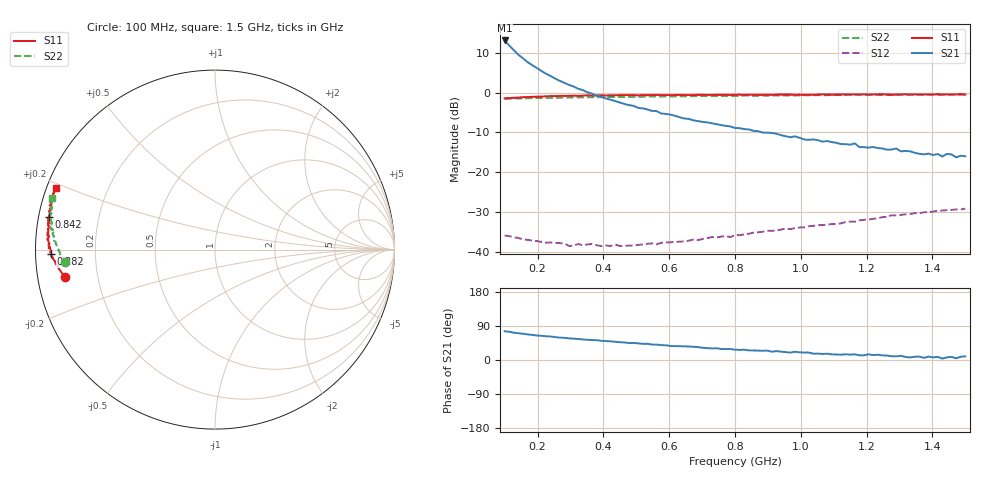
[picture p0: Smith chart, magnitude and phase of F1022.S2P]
!  POLYFET RF DEVICES
!  F1022
!  S PARAMETERS
!  VDS=28V, IDQ=600mA
! Date: Mon Oct 21 16:54:45 1991
! Bias (V mA) : V1=1.9979000  I1=0.0040389  V2=27.992500  I2=661.20100
# MHZ S MA R 50
!  FREQ  S11 MAG  S11 ANG  S21 MAG  S21 ANG  S12 MAG  S12 ANG  S22 MAG  S22 ANG
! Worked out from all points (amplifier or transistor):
!   101 points, 100 MHz to 1.5 GHz, reference 50 ohm
!   highest |S21| = 13.2 dB at 100 MHz (marker M1)
!   |S21| within 3 dB of that: start of sweep to 134.5 MHz
!   unconditionally stable (mu >= 1): 316.8 MHz to 343.9 MHz; 355.8 MHz to 1.444 GHz; 1.444 GHz to end of sweep
!   at 324 MHz: K = 1.04, MAG = 18.3 dB, |S12| = -38.1 dB
!   at 800 MHz: K = 1.65, MAG = 8.8 dB, |S12| = -35.8 dB
!   at 1.5 GHz: K = 1.10, MAG = 4.7 dB, |S12| = -29.2 dB
!   S11 on the Smith chart (normalised r, x): 100 MHz: 0.08, -0.09; 282 MHz: 0.05, -0.01; 842 MHz: 0.03, +0.10; 1.5 GHz: 0.03, +0.19
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100  0.8492 -169.5  4.552 76.0  0.0159 -5.0  0.8377 -175.2
114  0.8559 -170.5  3.932 74.5  0.01566 -3.9  0.8437 -175.3
128  0.8642 -171.4  3.43 72.0  0.01515 -3.5  0.843 -176.4
142  0.8698 -172.3  2.999 70.6  0.01485 -3.8  0.8485 -176.6
170  0.8805 -174.0  2.424 67.5  0.01405 -3.6  0.8522 -177.4
198  0.8917 -175.1  2.047 64.6  0.01357 -1.4  0.8571 -177.9
226  0.901 -176.4  1.732 62.6  0.01293 2.3  0.8637 -178.4
254  0.9048 -177.3  1.505 60.3  0.01285 1.4  0.8663 -179.0
282  0.9126 -178.4  1.33 58.4  0.01268 3.6  0.8707 -179.6
296  0.9146 -178.8  1.254 57.1  0.01175 5.4  0.8697 -179.8
338  0.9198 179.5  1.076 54.1  0.012 8.4  0.8757 179.7
380  0.9263 178.8  0.9142 52.2  0.01202 13.9  0.8786 179.1
450  0.9303 176.7  0.7534 46.9  0.01176 19.7  0.8868 178.0
576  0.9334 174.1  0.5467 39.1  0.01288 31.4  0.8957 176.1
800  0.9437 169.6  0.3603 27.3  0.01623 46.5  0.909 172.9
842  0.9437 168.9  0.3452 25.3  0.01678 50.0  0.9211 172.0
1038  0.9431 165.4  0.2588 16.6  0.02103 55.6  0.9312 169.4
1276  0.9459 162.1  0.1925 9.8  0.02868 61.0  0.9397 165.8
1430  0.9493 159.7  0.1574 3.7  0.03291 58.7  0.9454 163.7
1444  0.9537 159.4  0.17 7.0  0.03323 57.2  0.9478 163.4
1472  0.9548 158.8  0.1538 4.6  0.03394 57.2  0.9488 163.2
1500  0.9515 158.7  0.1586 9.7  0.03471 57.7  0.9496 162.5
